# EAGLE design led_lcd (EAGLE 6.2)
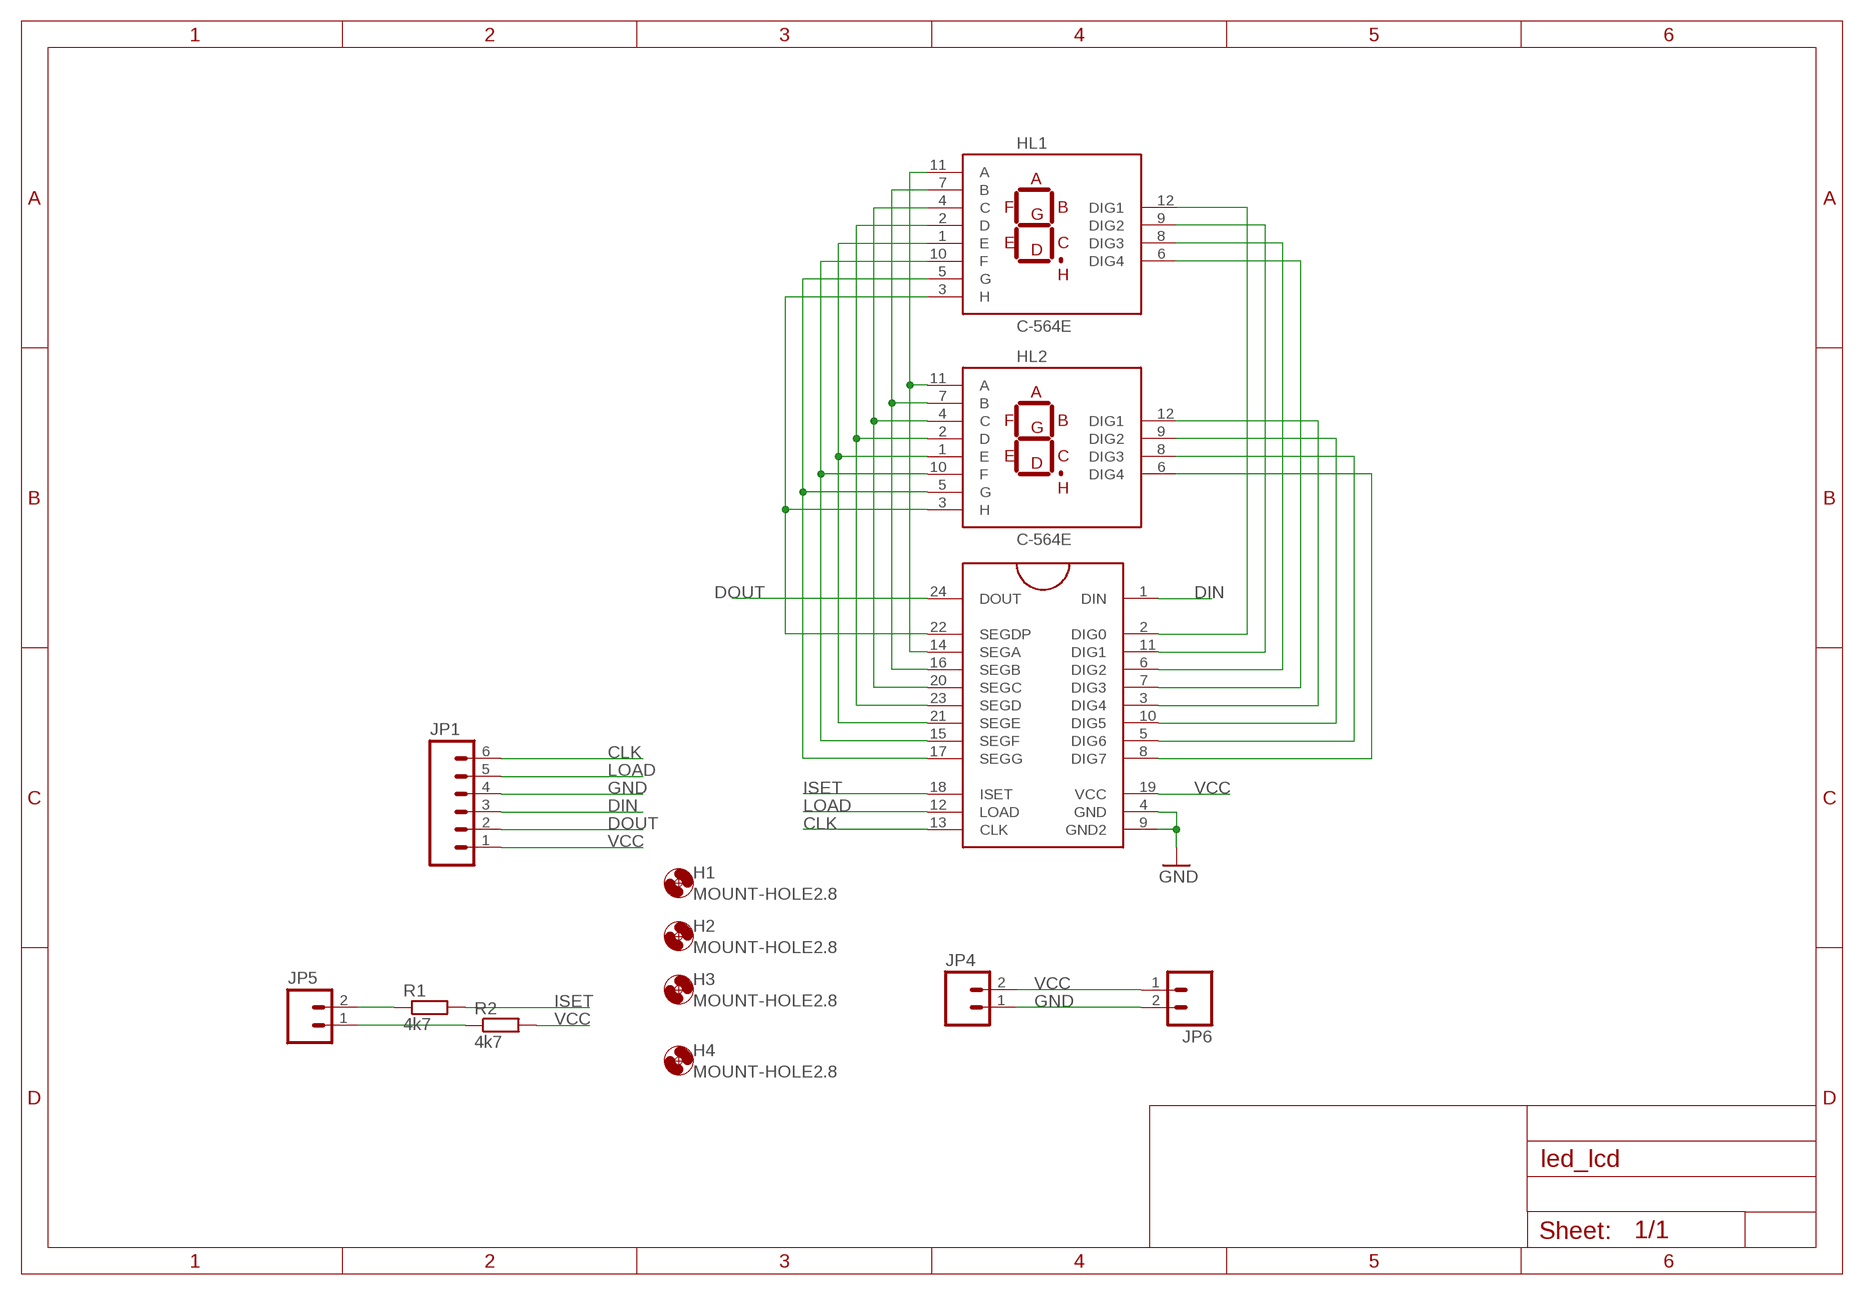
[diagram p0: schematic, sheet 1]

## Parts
H1  MOUNT-HOLE2.8  [2,8]
H2  MOUNT-HOLE2.8  [2,8]
H3  MOUNT-HOLE2.8  [2,8]
H4  MOUNT-HOLE2.8  [2,8]
HL1  C-564E  [C/A-564]
HL2  C-564E  [C/A-564]
JP1  M06LONGPADS  [1X06_LONGPADS]
JP4  M02LOCK_LONGPADS  [1X02_LOCK_LONGPADS]
JP5  M02LOCK_LONGPADS  [1X02_LOCK_LONGPADS]
JP6  M025MM  [SCREWTERMINAL-5MM-2]
R1  4k7  R-EU_R0805  [R0805]
R2  4k7  R-EU_R0805  [R0805]
U$1  MAX7219DIP  [DIL24]

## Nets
CLK: JP1.6 U$1.13(CLK)
DIN: JP1.3 U$1.1(DIN)
DOUT: JP1.2 U$1.24(DOUT)
GND: JP1.4 JP4.1 JP6.2 U$1.4(GND) U$1.9(GND2)
ISET: R1.2 U$1.18(ISET)
LOAD: JP1.5 U$1.12(LOAD)
N$1: HL1.11(A) HL2.11(A) U$1.14(SEGA)
N$2: HL1.7(B) HL2.7(B) U$1.16(SEGB)
N$3: HL1.4(C) HL2.4(C) U$1.20(SEGC)
N$4: HL1.2(D) HL2.2(D) U$1.23(SEGD)
N$5: HL1.1(E) HL2.1(E) U$1.21(SEGE)
N$6: HL1.10(F) HL2.10(F) U$1.15(SEGF)
N$7: HL1.5(G) HL2.5(G) U$1.17(SEGG)
N$8: HL1.3(H) HL2.3(H) U$1.22(SEGDP)
N$9: HL1.12(DIG1) U$1.2(DIG0)
N$10: HL1.9(DIG2) U$1.11(DIG1)
N$11: HL1.8(DIG3) U$1.6(DIG2)
N$12: HL1.6(DIG4) U$1.7(DIG3)
N$13: HL2.12(DIG1) U$1.3(DIG4)
N$14: HL2.9(DIG2) U$1.10(DIG5)
N$15: HL2.8(DIG3) U$1.5(DIG6)
N$16: HL2.6(DIG4) U$1.8(DIG7)
N$17: JP5.2 R1.1
N$18: JP5.1 R2.1
VCC: JP1.1 JP4.2 JP6.1 R2.2 U$1.19(VCC)

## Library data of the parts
H1-H4 = holes:MOUNT-HOLE: MOUNTING HOLE with drill center marker
HL1 HL2 = led7seg:C-564: Para Light C-564x Four digits 7seg display Common cathode. 50x19 mm place. 14.22mm (560 mil) digit height 2009 Draw by Ivan A-R. License CC-BY-SA 3.0
JP1 = SparkFun:M06: Header 6 Standard 6-pin 0.1" header. Use with straight break away headers (SKU : PRT-00116), right angle break away headers (PRT-00553), swiss pins (PRT-00743), machine pins (PRT-00117), and female headers (PRT-00115). Molex polarized connector foot print use with SKU : PRT-08094 with associated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
JP4-JP6 = SparkFun:M02: Header 2
R1 R2 = rcl:R-EU_: RESISTOR, European symbol
U$1 = SparkFun:MAX7219

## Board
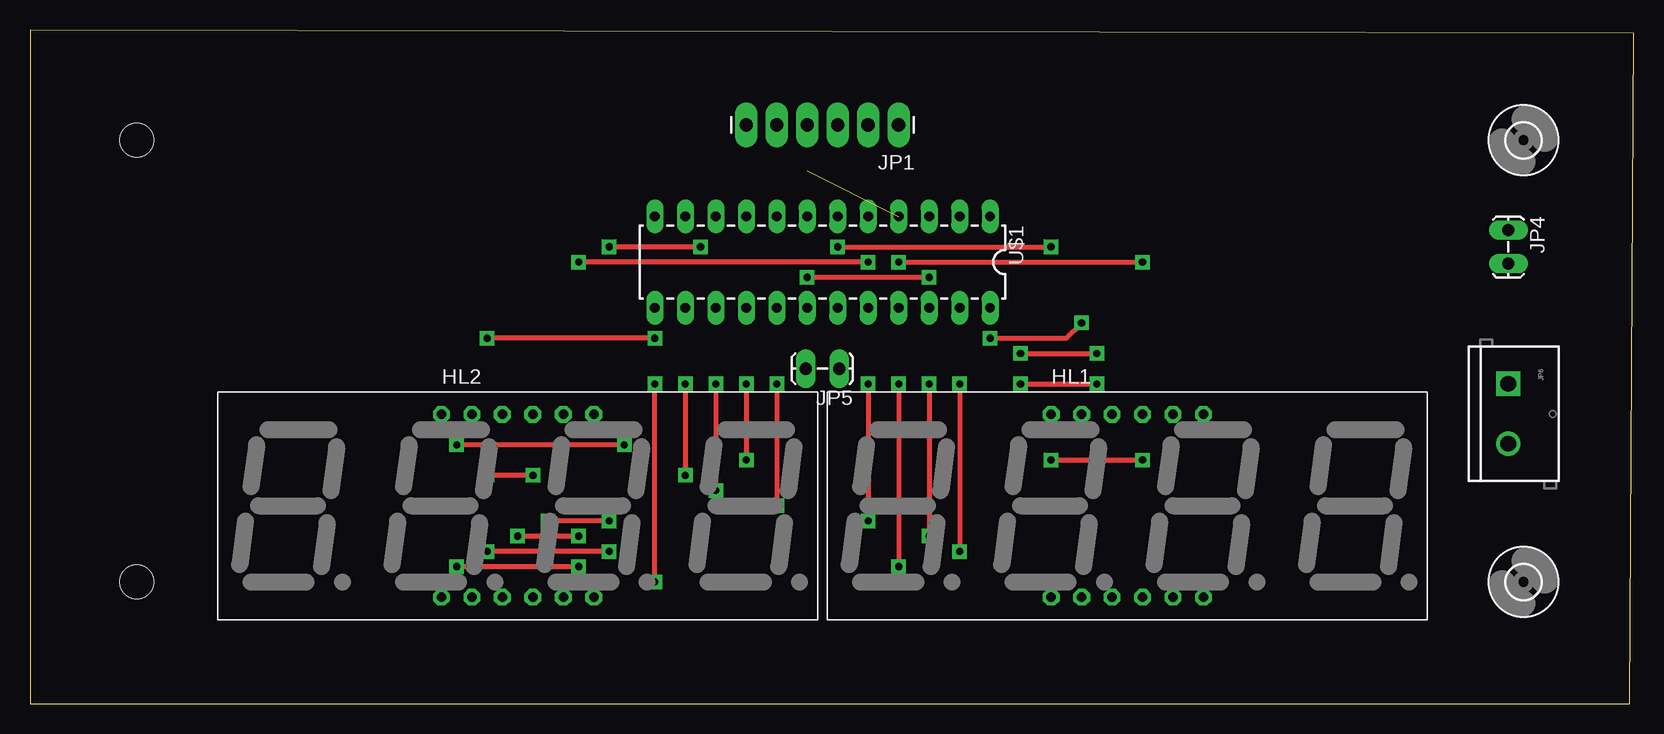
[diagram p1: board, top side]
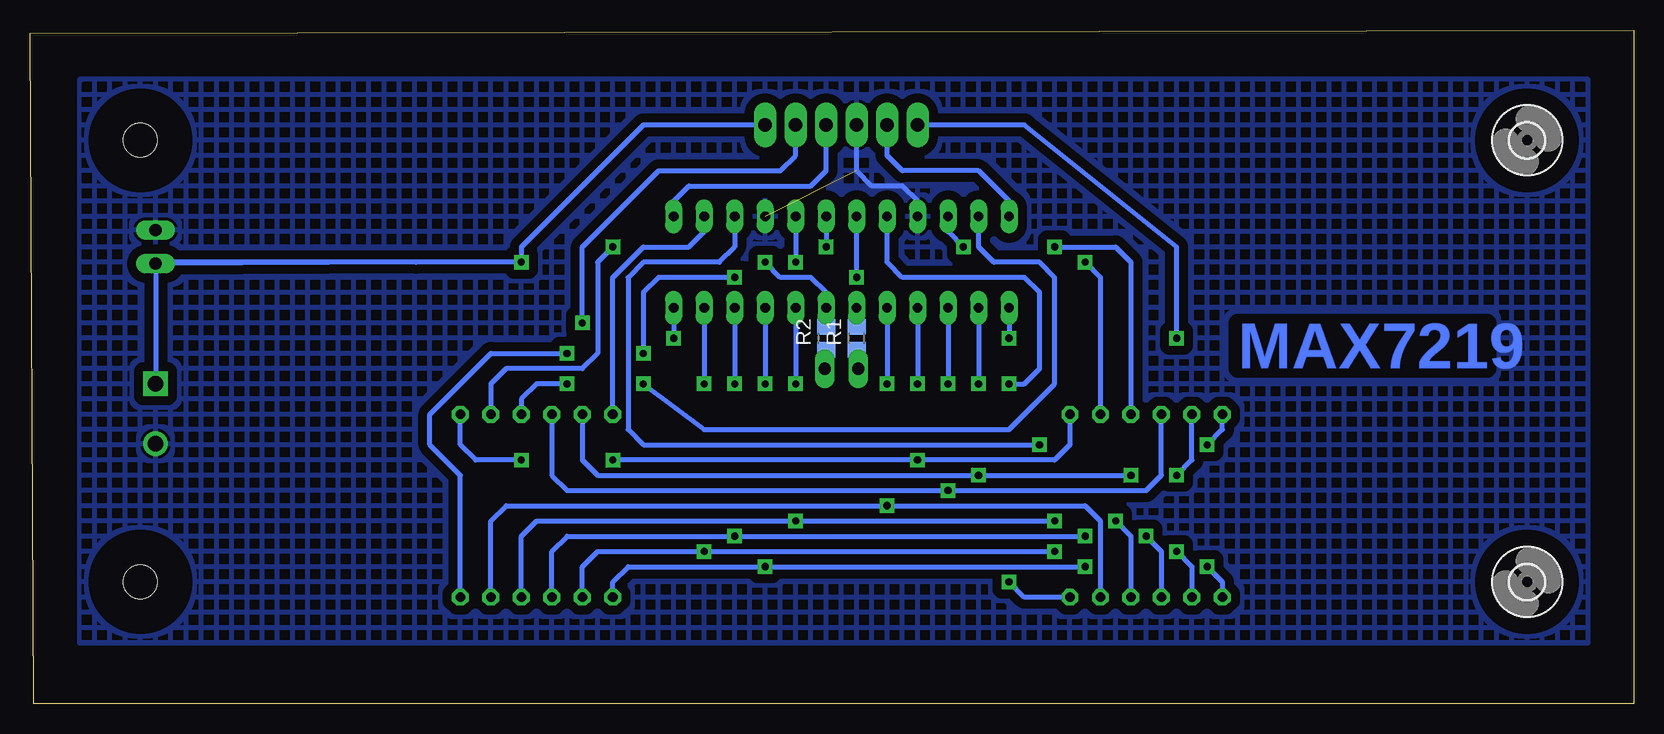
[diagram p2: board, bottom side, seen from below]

Size 133.66 x 56.19 mm. Coordinates in mm from the lower left corner, seen from the top.
Outline: 0,0 133.33,0 133.66,55.9 0,56.19 0,0
Copper layers (1*16): Top 0.035mm / dielectric 1.5mm / Bottom 0.035mm
Design rules: minimum track width 10mil, minimum drill 32mil, track to track 12mil, track to pad 12mil, pad to pad 12mil, via to via 12mil, smd to smd 8mil, copper to edge 40mil, drill to drill 40mil, minimum pad ring 12mil, minimum via ring 12mil, stop-mask expansion 4mil, vias tented up to drill 0mil, thermal gap 10mil

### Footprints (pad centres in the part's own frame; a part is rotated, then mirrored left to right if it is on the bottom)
2,8 = hole 2.8: 0,0
C/A-564 = drill 0.8 octagon: 1 -6.35,-7.62; 2 -3.81,-7.62; 3 -1.27,-7.62; 4 1.27,-7.62; 5 3.81,-7.62; 6 6.35,-7.62; 7 6.35,7.62; 8 3.81,7.62; 9 1.27,7.62; 10 -1.27,7.62; 11 -3.81,7.62; 12 -6.35,7.62
1X06_LONGPADS = drill 1.118 pad 1.88 long: 1 0,0; 2 2.54,0; 3 5.08,0; 4 7.62,0; 5 10.16,0; 6 12.7,0
1X02_LOCK_LONGPADS = drill 1.016 long: 1 -0.127,0; 2 2.667,0
SCREWTERMINAL-5MM-2 = drill 1.3 pad 2.032 square: 1 0,0 | drill 1.3 pad 2.032: 2 5,0
R0805 = smd 1.3 x 1.5: 1 -0.95,0; 2 0.95,0
DIL24 = drill 0.813 long: 1 -13.97,-3.81; 2 -11.43,-3.81; 3 -8.89,-3.81; 4 -6.35,-3.81; 5 -3.81,-3.81; 6 -1.27,-3.81; 7 1.27,-3.81; 8 3.81,-3.81; 9 6.35,-3.81; 10 8.89,-3.81; 11 11.43,-3.81; 12 13.97,-3.81; 13 13.97,3.81; 14 11.43,3.81; 15 8.89,3.81; 16 6.35,3.81; 17 3.81,3.81; 18 1.27,3.81; 19 -1.27,3.81; 20 -3.81,3.81; 21 -6.35,3.81; 22 -8.89,3.81; 23 -11.43,3.81; 24 -13.97,3.81

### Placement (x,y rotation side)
H1  124.46,10.16 0 top
H2  8.89,46.99 0 bottom
H3  8.89,10.16 0 bottom
H4  124.46,46.99 0 top
HL1  91.44,16.51 0 top
HL2  40.64,16.51 0 top
JP1  72.39,48.26 180 top
JP4  123.19,39.37 270 top
JP5  67.31,27.94 180 top
JP6  123.19,26.67 270 top
R1  64.77,30.48 90 bottom
R2  67.31,30.48 90 bottom
U$1  66.04,36.83 180 top

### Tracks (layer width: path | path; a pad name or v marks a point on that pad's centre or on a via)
CLK  (via drill 0.6)
  Top 0.406: v52.07,30.48 v38.1,30.48
  Bottom 0.406: U$1.13 v52.07,30.48 | v38.1,30.48 38.1,38.1 50.8,48.26 JP1.6
DIN
  Bottom 0.406: U$1.1 80.01,41.91 78.74,43.18 68.58,43.18 67.31,44.45 JP1.3
DOUT  (via drill 0.6)
  Top 0.406: v80.01,30.48 86.36,30.48 v87.63,31.75
  Bottom 0.406: U$1.24 v80.01,30.48 | v87.63,31.75 87.63,38.1 81.28,44.45 71.12,44.45 69.85,45.72 JP1.2
GND  (1 unrouted)
  Bottom 0.406: U$1.9 59.69,41.91 60.96,43.18 63.5,43.18 64.77,44.45 JP1.4
  pour Bottom (isolate 0.762, hatched): 3.81,52.07 129.54,52.07 129.54,5.08 3.81,5.08
ISET
  Bottom 0.406: U$1.18 R1.2
LOAD
  Bottom 0.406: U$1.12 52.07,41.91 54.61,44.45 60.96,44.45 62.23,45.72 JP1.5
N$1  (via drill 0.6)
  Top 0.406: v41.91,19.05 v38.1,19.05 | v54.61,26.67 v54.61,19.05
  Bottom 0.406: HL1.11 87.63,20.32 86.36,19.05 v54.61,19.05 v41.91,19.05 | v38.1,19.05 36.83,20.32 HL2.11 | U$1.14 v54.61,26.67
N$2  (via drill 0.6)
  Top 0.406: v85.09,20.32 v92.71,20.32 | v59.69,26.67 v59.69,20.32
  Bottom 0.406: HL2.7 46.99,21.59 48.26,20.32 v59.69,20.32 v85.09,20.32 | v92.71,20.32 96.52,20.32 97.79,21.59 HL1.7 | U$1.16 v59.69,26.67
N$3  (via drill 0.6)
  Top 0.406: v69.85,26.67 v69.85,15.24 | v48.26,15.24 v43.18,15.24
  Bottom 0.406: HL1.4 92.71,13.97 91.44,15.24 v69.85,15.24 v48.26,15.24 | v43.18,15.24 41.91,13.97 HL2.4 | U$1.20 v69.85,26.67
N$4  (via drill 0.6)
  Top 0.406: v77.47,26.67 v77.47,12.7 | v48.26,12.7 v38.1,12.7
  Bottom 0.406: HL1.2 87.63,11.43 86.36,12.7 v77.47,12.7 v48.26,12.7 | v38.1,12.7 36.83,11.43 HL2.2 | U$1.23 v77.47,26.67
N$5  (via drill 0.6)
  Top 0.406: v72.39,26.67 v72.39,11.43 | v45.72,11.43 v35.56,11.43
  Bottom 0.406: v35.56,11.43 34.29,10.16 HL2.1 | U$1.21 v72.39,26.67 | HL1.1 85.09,10.16 83.82,11.43 v72.39,11.43 v45.72,11.43
N$6  (via drill 0.6)
  Top 0.406: v57.15,26.67 v57.15,17.78
  Bottom 0.406: HL1.10 90.17,19.05 88.9,17.78 v57.15,17.78 40.64,17.78 39.37,19.05 HL2.10 | U$1.15 v57.15,26.67
N$7  (via drill 0.6)
  Top 0.406: v62.23,26.67 v62.23,16.51
  Bottom 0.406: HL1.5 95.25,15.24 93.98,16.51 v62.23,16.51 45.72,16.51 44.45,15.24 HL2.5 | U$1.17 v62.23,26.67
N$8  (via drill 0.6)
  Top 0.406: v74.93,26.67 v74.93,13.97 | v45.72,13.97 v40.64,13.97
  Bottom 0.406: HL1.3 90.17,12.7 88.9,13.97 v74.93,13.97 v45.72,13.97 | v40.64,13.97 39.37,12.7 HL2.3 | U$1.22 v74.93,26.67
N$9
  Bottom 0.406: HL1.12 85.09,35.56 82.55,38.1 78.74,38.1 77.47,39.37 U$1.2
N$10  (via drill 0.6)
  Top 0.406: v82.55,26.67 v88.9,26.67
  Bottom 0.406: v88.9,26.67 91.44,26.67 92.71,25.4 HL1.9 | v82.55,26.67 77.47,22.86 52.07,22.86 48.26,26.67 48.26,35.56 49.53,36.83 53.34,36.83 54.61,38.1 U$1.11
N$11  (via drill 0.6)
  Top 0.406: v67.31,38.1 v85.09,38.1
  Bottom 0.406: U$1.6 v67.31,38.1 | v85.09,38.1 86.36,36.83 86.36,29.21 87.63,27.94 93.98,27.94 95.25,26.67 HL1.8
N$12  (via drill 0.6)
  Top 0.406: v74.93,35.56 v64.77,35.56 | v82.55,29.21 v88.9,29.21
  Bottom 0.406: HL1.6 97.79,19.05 100.33,21.59 100.33,24.13 95.25,29.21 v88.9,29.21 | v64.77,35.56 U$1.7 | v74.93,35.56 81.28,35.56 82.55,34.29 v82.55,29.21
N$13  (via drill 0.6)
  Top 0.406: v49.53,21.59 v35.56,21.59
  Bottom 0.406: U$1.3 74.93,38.1 76.2,36.83 82.55,36.83 83.82,35.56 83.82,22.86 82.55,21.59 v49.53,21.59 | v35.56,21.59 34.29,22.86 HL2.12
N$14  (via drill 0.6)
  Top 0.406: v55.88,38.1 v48.26,38.1
  Bottom 0.406: U$1.10 57.15,39.37 v55.88,38.1 | v48.26,38.1 43.18,38.1 41.91,36.83 HL2.9
N$15  (via drill 0.6)
  Top 0.406: v69.85,36.83 v45.72,36.83
  Bottom 0.406: U$1.5 v69.85,36.83 | v45.72,36.83 44.45,35.56 HL2.8
N$16  (via drill 0.6)
  Top 0.406: v52.07,10.16 v52.07,26.67
  Bottom 0.406: HL2.6 50.8,8.89 v52.07,10.16 | v52.07,26.67 50.8,26.67 49.53,27.94 49.53,34.29 50.8,35.56 60.96,35.56 62.23,36.83 U$1.8
N$17
  Bottom 0.406: JP5.2 64.64,29.4 R1.1
N$18
  Bottom 0.406: JP5.1 67.44,29.4 R2.1
VCC  (via drill 0.6)
  Top 0.406: v72.39,36.83 v92.71,36.83
  Bottom 0.406: v72.39,36.83 71.12,35.56 68.58,35.56 67.31,34.29 U$1.19 R2.2 | 101.47,36.83 v92.71,36.83 92.71,38.1 82.55,48.26 JP1.1 | 101.47,36.83 JP4.2 | 101.47,36.83 123.19,36.83 JP6.1

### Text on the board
Bottom: MAX7219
